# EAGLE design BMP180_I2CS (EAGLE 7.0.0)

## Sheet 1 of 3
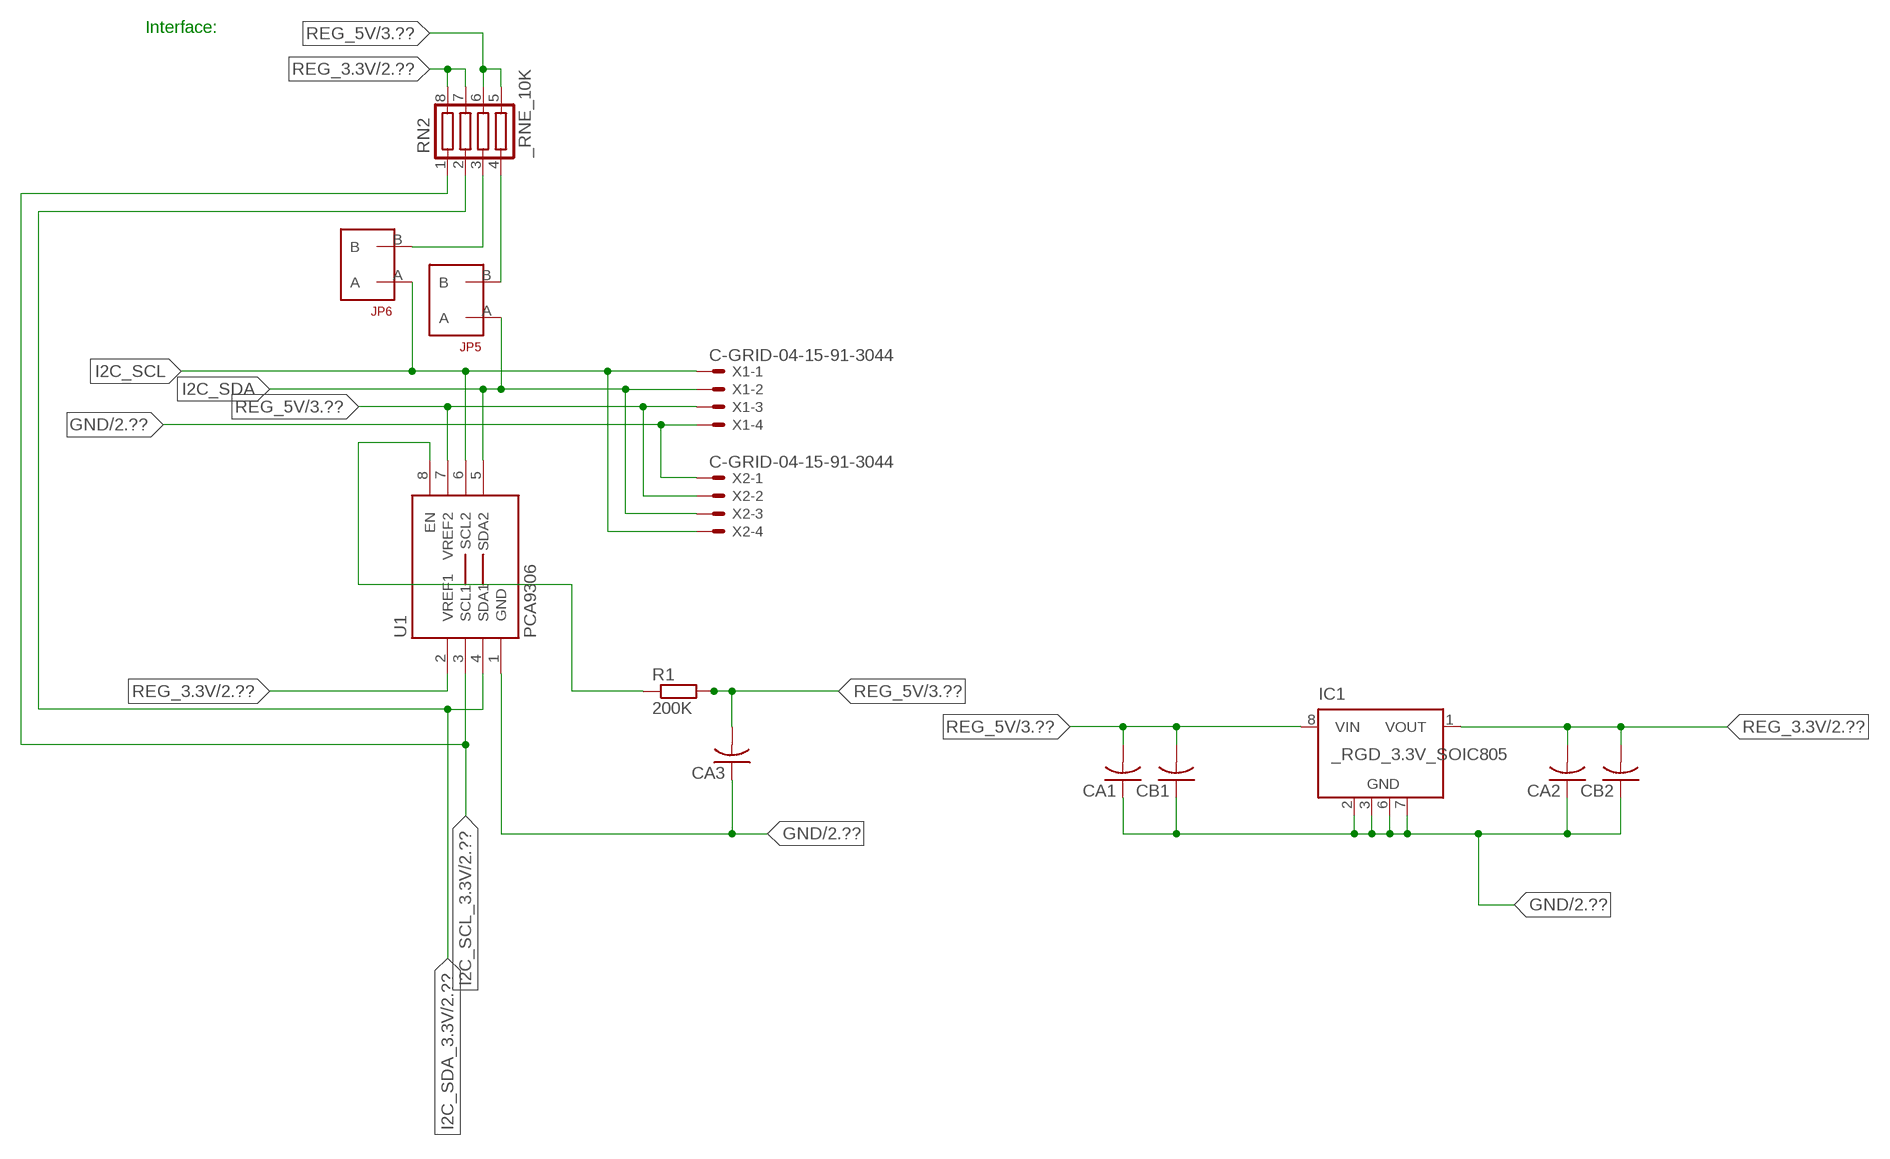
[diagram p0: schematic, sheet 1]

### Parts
CA1  CC1206KRX7R9BB104  [.1UF]
CA2  CC1206KRX7R9BB104  [.1UF]
CA3  CC1206KRX7R9BB104  [.1UF]
CB1  TMK316F106ZL-TC1206K  [TMK316F106ZL-T]
CB2  TMK316F106ZL-TC1206K  [TMK316F106ZL-T]
IC1  _RGD_3.3V_SOIC805  [_RGC_3.3V_SOIC8]
JP5  JUMPER_1X2_2MM  [JUMPER_1X2_2MM]
JP6  JUMPER_1X2_2MM  [JUMPER_1X2_2MM]
R1  200K  RESISTOR_SMT-0603  [R603]
RN2  _RNE_10K  [RNE]
U1  PCA9306  PCA9306_NCD  [PSOP-8]
X1  C-GRID-04-15-91-3044  [15-91-04]
X2  C-GRID-04-15-91-3044  [15-91-04]

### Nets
GND: CA1.1 CA2.1 CA3.1 CB1.1 CB2.1 IC1.2(GND) IC1.3(GND) IC1.6(GND) IC1.7(GND) U1.1(GND) X1.4 X2.1 ; also sheet 2,3
I2C_SCL: JP6.A U1.6(SCL2) X1.1 X2.4
I2C_SCL_3.3V: RN2.1 U1.3(SCL1) ; also sheet 2
I2C_SDA: JP5.A U1.5(SDA2) X1.2 X2.3
I2C_SDA_3.3V: RN2.2 U1.4(SDA1) ; also sheet 2
N$1: JP6.B RN2.3
N$2: JP5.B RN2.4
N$23: R1.1 U1.8(EN)
REG_3.3V: CA2.2 CB2.2 IC1.1(VOUT) RN2.7 RN2.8 U1.2(VREF1) ; also sheet 2
REG_5V: CA1.2 CA3.2 CB1.2 IC1.8(VIN) R1.2 RN2.5 RN2.6 U1.7(VREF2) X1.3 X2.2 ; also sheet 3
Unconnected: IC1.4(NC) IC1.5(NC)

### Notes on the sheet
- Interface:

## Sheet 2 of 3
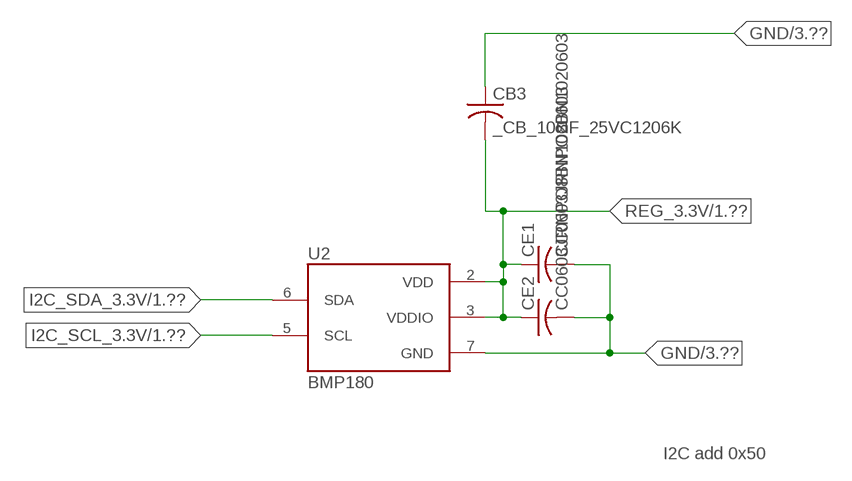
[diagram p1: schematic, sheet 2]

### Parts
CB3  _CB_10UF_25VC1206K  [_CB_10UF_25V]
CE1  CC0603JRNPO8BN1020603  [CC0603JRNPO8BN102]
CE2  CC0603JRNPO8BN1020603  [CC0603JRNPO8BN102]
U2  BMP180  [BMP180]

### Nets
GND: CB3.1 CE1.2 CE2.2 U2.7(GND) ; also sheet 1,3
I2C_SCL_3.3V: U2.5(SCL) ; also sheet 1
I2C_SDA_3.3V: U2.6(SDA) ; also sheet 1
REG_3.3V: CB3.2 CE1.1 CE2.1 U2.2(VDD) U2.3(VDDIO) ; also sheet 1

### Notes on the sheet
- I2C add 0x50

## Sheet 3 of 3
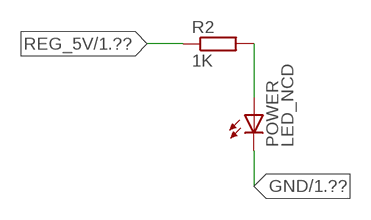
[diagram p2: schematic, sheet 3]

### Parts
POWER  LED_NCD  [CHIPLED_0603]
R2  1K  RESISTOR_SMT-0402  [R402]

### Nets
GND: POWER.C ; also sheet 1,2
N$4: POWER.A R2.2
REG_5V: R2.1 ; also sheet 1

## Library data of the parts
CA1-CA3 = NCD_ULTIMATE_LIBRARY:CC1206KRX7R9BB104: Capacitor CA .1uF 50V SMT C1206K CC1206KRX7R9BB104
CB1 CB2 = NCD_ULTIMATE_LIBRARY:TMK316F106ZL-T: Capacitor CB 10uF SMT 1206 TMK316F106ZL-T
CB3 = NCD_ULTIMATE_LIBRARY:_CB_10UF_25V: Capacitor 10uF SMT
CE1 CE2 = NCD_ULTIMATE_LIBRARY:CC0603JRNPO8BN102: Capacitor CE 1uF SMT CC0603JRNPO8BN102 0603
IC1 = NCD_ULTIMATE_LIBRARY:_RGD_3.3V_SOIC8: Regulator Linear 3.3V Chip Positive VOLTAGE REGULATOR Digikey 497-1199-2-ND/L78L33ACD13TR
JP5 JP6 = NCD_ULTIMATE_CONNECTORS:JUMPER_1X2_2MM
POWER = NCD_ULTIMATE_LIBRARY:LED_NCD: LED Digikey 754-1132-2-ND/APT2012SRCPRV
R1 R2 = NCD_ULTIMATE_LIBRARY:RESISTOR_SMT: NCD Resistor
RN2 = NCD_ULTIMATE_LIBRARY:_RNE_10K: Resistor Array RNE SMT 10K x 4 Single Resistor Source: http://www.ctscorp.com/components/Datasheets/CTSChipArrayDs.pdf Digikey 742C083103JPTR-ND/742C083103JP; OC_FARNELL: unknown; OC_NEWARK: unknown
U1 = NCD_ULTIMATE_LIBRARY:PCA9306_NCD: NCD Bidirectional I2C level shifter. NOT compatible with all available part number pinout schemes- DOUBLE CHECK!!!; PROD_ID: IC-10023
U2 = NCD_ULTIMATE_bhaskar:BMP180: BOSCH BMP180 DIGITAL BAROMETRIC PRESSURE SENSOR Web page: http://www.bosch-sensortec.com/en/homepage/products_3/environmental_sensors_1/bmp180_1/bmp180 Datasheet: http://ae-bst.resource.bosch.com/media/products/dokumente/bmp180/BST-BMP180-DS000-09.pdf The BMP180 is the function compatible successor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
X1 X2 = NCD_ULTIMATE_CONNECTORS:C-GRID-04: CONNECTOR 4-Pos I2C wire to board 2.54 mm (0.100") pitch header Digikey WM1342-ND/0015912045; OC_FARNELL: unknown; OC_NEWARK: unknown

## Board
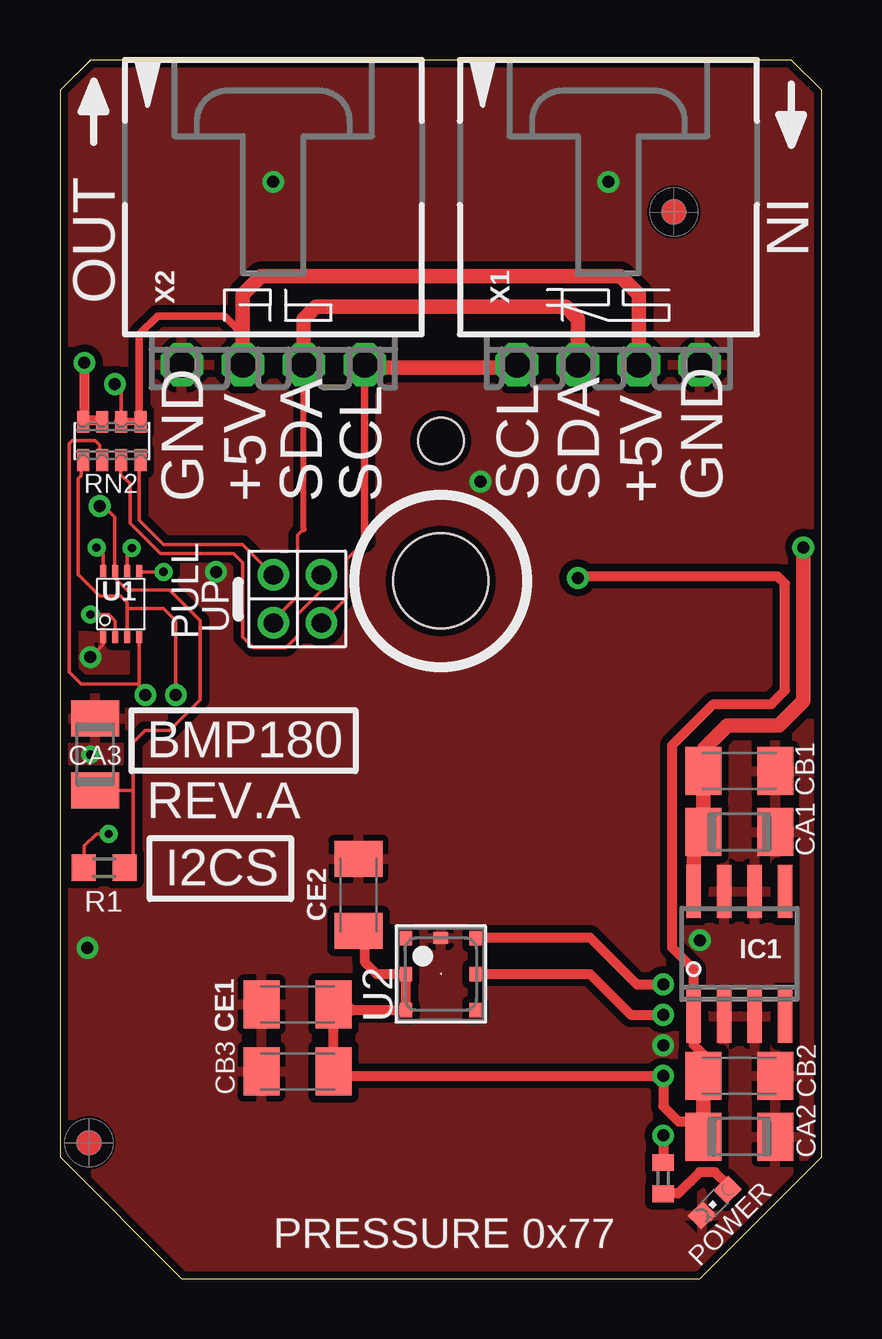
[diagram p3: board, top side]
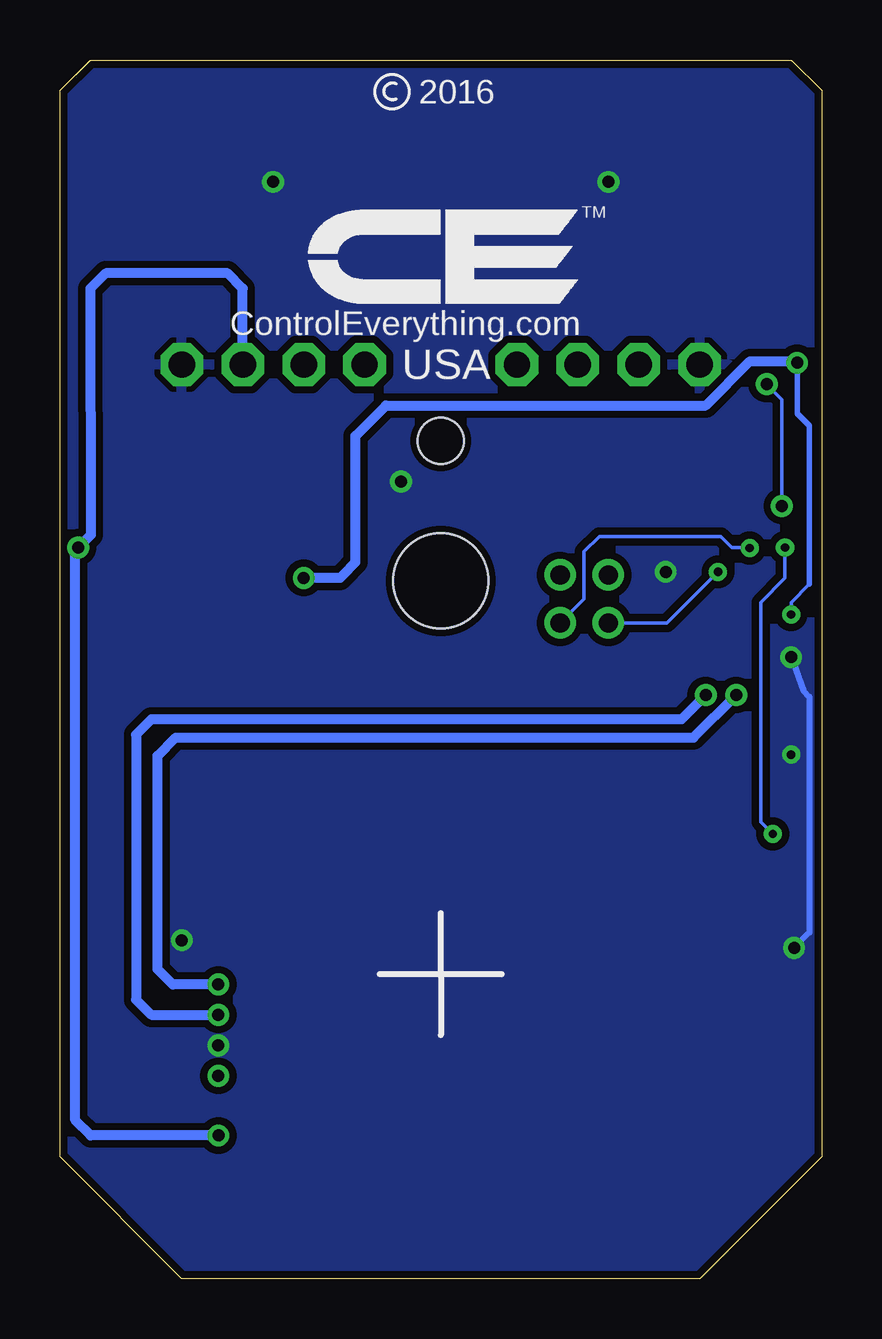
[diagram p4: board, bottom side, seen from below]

Size 31.75 x 50.8 mm. Coordinates in mm from the lower left corner, seen from the top.
Outline: 48 segments
Copper layers (1*16): Top 0.035mm / dielectric 1.5mm / Bottom 0.035mm
Design rules "default": minimum track width 5mil, minimum drill 24mil, track to track 5mil, track to pad 5mil, pad to pad 5mil, via to via 5mil, smd to smd 5mil, copper to edge 10mil, drill to drill 8mil, minimum pad ring 10mil, minimum via ring 8mil, stop-mask expansion 2mil, vias tented up to drill 0mil, thermal gap 10mil
Holes 3.96 mm at 15.88,29.08
Holes 1.91 mm at 15.88,34.93

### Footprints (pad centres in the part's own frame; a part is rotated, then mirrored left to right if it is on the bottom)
.1UF = smd 1.5 x 2: 1 -1.5,0; 2 1.5,0
TMK316F106ZL-T = smd 1.5 x 2: 1 -1.5,0; 2 1.5,0
_CB_10UF_25V = smd 1.5 x 2: 1 -1.5,0; 2 1.5,0
CC0603JRNPO8BN102 = smd 1.5 x 2: 1 -1.5,0; 2 1.5,0
_RGC_3.3V_SOIC8 = smd 0.6 x 2.2: 1 -1.905,-2.6; 2 -0.635,-2.6; 3 0.635,-2.6; 4 1.905,-2.6; 5 1.905,2.6; 6 0.635,2.6; 7 -0.635,2.6; 8 -1.905,2.6
JUMPER_1X2_2MM = drill 0.8: A 0,2; B 0,0
CHIPLED_0603 = smd 0.8 x 0.876: A 0,-0.75; C 0,0.75
R603 = smd 1 x 1.1: 1 -0.85,0; 2 0.85,0
R402 = smd 0.7 x 0.9: 1 -0.65,0; 2 0.65,0
RNE = smd 0.5 x 0.9: 1 -1.2,-0.8; 2 -0.4,-0.8; 3 0.4,-0.8; 4 1.2,-0.8; 5 1.2,0.8; 6 0.4,0.8; 7 -0.4,0.8; 8 -1.2,0.8
PSOP-8 = smd 0.25 x 0.5: 1 -0.73,-1.37; 2 -0.23,-1.37; 3 0.27,-1.37; 4 0.77,-1.37; 5 0.77,1.38; 6 0.27,1.38; 7 -0.23,1.38; 8 -0.73,1.38
BMP180 = smd 0.6 x 0.5: 1 1.5,1.45; 2 0,1.45; 3 -1.5,1.45; 4 -1.5,-1.45; 5 0,-1.45; 6 1.5,-1.45 | smd 0.5 x 0.6: 7 1.5,0
15-91-04 = drill 1.1 pad 1.778 octagon: 1 -3.81,-7.62; 2 -1.27,-7.62; 3 1.27,-7.62; 4 3.81,-7.62

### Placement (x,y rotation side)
CA1  28.32,18.62 180 top
CA2  28.32,5.92 180 top
CA3  1.46,21.86 270 top
CB1  28.32,21.16 180 top
CB2  28.32,8.46 180 top
CB3  9.91,8.64 0 top
CE1  9.91,11.43 180 top
CE2  12.45,16 90 top
IC1  28.32,13.54 0 top
JP5  8.89,29.34 180 top
JP6  10.9,29.34 180 top
POWER  27.3,3.18 135 top
R1  1.84,17.13 0 top
R2  25.15,4.19 270 top
RN2  2.16,34.93 0 top
U1  2.54,28.12 0 top
U2  15.88,12.7 90 top
U$5  [VISION_REF10]  1.21,5.66 90 top
U$28  [VISION_REF10]  25.59,44.46 90 top
X1  22.86,45.72 0 top
X2  8.89,45.72 0 top

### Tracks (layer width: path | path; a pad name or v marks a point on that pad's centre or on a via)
GND  (via drill 0.35, 0.5)
  Top 0.152: CA3.1 1.52,23.42 1.52,23.62 | v1.27,25.91 1.81,26.45 U1.1
  Bottom 0.254: v1.27,25.91 0.76,24.51 0.51,24.26 0.51,14.43 v1.15,13.79
  other vias: 8.89,45.72 22.86,45.72 25.15,9.73 17.53,33.22 26.67,14.11 6.5,29.46 1.27,21.84
  pour Bottom (isolate 0.305): -0.64,5.08 -0.64,49.53 1.27,51.44 30.48,51.44 32.38,49.53 32.38,5.08 26.67,-0.63 5.08,-0.63
  pour Top (isolate 0.305): 4.45,-1.27 -1.27,4.45 -1.27,50.17 0.64,52.07 31.11,52.07 33.02,50.17 33.02,4.45 27.3,-1.27
I2C_SCL  (via drill 0.35)
  Top 0.152: 12.7,30.73 11.94,29.97 11.94,28.38 JP6.A | v3,30.46 2.81,30.24 U1.6
  Top 0.305: 12.7,30.73 X2.4
  Top 0.406: X2.4 12.7,37.97 | 19.05,37.97 X1.1
  Top 0.61: 12.7,37.97 19.05,37.97
  Bottom 0.152: JP6.A 9.91,28.33 9.91,30.3 9.27,30.94 4.19,30.94 3.74,30.48 3.02,30.48 v3,30.46
I2C_SCL_3.3V  (via drill 0.5)
  Top 0.152: RN2.1 0.89,34.07 0.89,33.48 0.77,33.35 0.77,29.35 1.67,28.45 2.54,28.45 2.81,28.18 2.81,27.94 | 2.81,27.94 U1.3 | v4.83,24.33 v4.83,24.34 4.83,27.43 4.32,27.94 2.81,27.94
  Top 0.406: U2.5 22.1,12.7 23.8,11 v25.15,11
  Bottom 0.406: v4.83,24.33 5.84,23.32 27.94,23.32 28.58,22.68 28.58,11.63 27.94,11 v25.15,11
I2C_SDA  (via drill 0.35)
  Top 0.152: JP5.A 8.89,27.44 9.91,28.45 9.91,30.99 10.16,31.24 | U1.5 3.34,29.46 v4.32,29.46
  Top 0.254: 10.16,31.24 10.16,31.25 X2.3
  Top 0.61: X2.3 10.16,40.01 10.67,40.51 21.09,40.51 21.59,40.01 X1.2
  Bottom 0.152: v4.32,29.46 6.45,27.34 JP5.A
I2C_SDA_3.3V  (via drill 0.5)
  Top 0.152: RN2.2 1.65,34.14 1.65,34.75 1.46,34.94 0.51,34.94 0.38,34.81 0.38,26.37 0.38,26.36 0.38,25.3 0.89,24.79 3.31,24.79 | v3.56,24.33 3.31,24.58 3.31,24.79 | 3.31,24.79 U1.4
  Top 0.406: U2.6 17.48,14.22 22.1,14.22 24.05,12.27 v25.15,12.27
  Bottom 0.406: v25.15,12.27 27.05,12.27 27.69,12.9 27.69,21.79 26.93,22.56 5.34,22.56 v3.56,24.33
N$1
  Top 0.152: JP6.B 10.92,29.31 10.92,28.7 9.91,27.69 9.91,26.8 9.42,26.31 8.06,26.31 7.62,26.75 7.62,29.84 7.24,30.23 4.19,30.23 2.92,31.5 2.92,33.15 2.54,33.53 2.54,34.1 RN2.3
  Top 0.305: 2.54,34.02 RN2.3
N$2
  Top 0.152: JP5.B 7.62,30.61 4.32,30.61 3.3,31.62 3.3,34.07 RN2.4
  Top 0.305: 3.37,33.88 RN2.4
N$4
  Top 0.406: POWER.A 27.84,3.92 27.3,4.45 26.67,4.45 25.78,3.56 25.16,3.56 R2.2
N$23  (via drill 0.35)
  Top 0.152: R1.1 1.02,17.16 1.02,18.03 1.52,18.54 v2.03,18.54 | v1.52,30.48 1.81,30.2 U1.8
  Bottom 0.152: v2.03,18.54 2.54,19.05 2.54,28.19 1.52,29.21 v1.52,30.48
REG_3.3V  (via drill 0.35, 0.5)
  Top 0.152: v1.27,27.69 2.03,27.69 2.31,27.41 U1.2
  Top 0.406: CB2.2 26.82,9.35 26.42,9.75 26.42,10.36 | 26.82,6.55 25.78,6.55 25.15,7.19 v25.15,8.46 11.58,8.46 CB3.2 CE1.1 11.94,11.43 12.19,11.18 14.53,11.18 U2.3 U2.2 13.21,12.7 12.7,13.21 12.7,14.25 CE2.1 | IC1.1 26.42,12.9 25.53,13.79 25.53,22.24 27.24,23.95 29.66,23.95 30.23,24.52 30.23,28.97 29.91,29.29 21.67,29.29 v21.59,29.21 | 26.52,5.62 CA2.2 | v1.02,38.18 1.02,35.78 | 1.02,35.78 RN2.8 | 1.02,35.78 1.71,35.78 RN2.7
  Top 0.61: CB2.2 26.82,6.55 CA2.2 | 26.42,10.36 IC1.1
  Bottom 0.152: 0.51,28.96 1.27,28.19 v1.27,27.69
  Bottom 0.229: 0.51,28.96 0.51,35.56 1.02,36.07 v1.02,38.18
  Bottom 0.406: v1.02,38.18 1.08,38.24 2.99,38.24 4.83,36.4 18.16,36.4 19.43,35.13 19.43,29.87 19.94,29.34 20.07,29.21 v21.59,29.21
REG_5V  (via drill 0.5)
  Top 0.152: RN2.6 2.56,37.01 v2.29,37.29 | R1.2 3.05,17.49 3.05,20.36 | 3.05,20.36 3.05,22.35 3.56,22.86 4.57,22.86 5.84,24.13 5.84,27.43 4.57,28.7 2.79,28.7 2.31,29.19 U1.7 2.29,29.52 2.29,31.75 1.83,32.21 v1.65,32.21 | CA3.2 3.05,20.36
  Top 0.305: 7.62,39.37 7.5,39.37 | 2.42,35.74 RN2.6 RN2.5 3.31,35.8 3.31,39.37 4.07,40.13 6.86,40.13 7.62,39.37 | X2.2 7.62,39.37
  Top 0.406: v25.15,5.97 R2.1
  Top 0.61: X2.2 7.62,41.02 8.38,41.78 23.37,41.78 24.13,41.02 X1.3 | IC1.8 26.42,18.21 CA1.2 CB1.2 26.86,21.2 26.86,22.11 27.82,23.06 29.98,23.06 30.99,24.08 v30.99,30.48
  Bottom 0.152: v1.65,32.21 1.65,36.65 v2.29,37.29
  Bottom 0.406: X1.3 24.13,41.28 24.77,41.91 29.84,41.91 30.48,41.27 30.47,31 v30.99,30.48 31.11,30.36 31.11,6.6 30.48,5.97 v25.15,5.97

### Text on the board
tNames: IN | OUT | GND | +5V | SDA | SCL | SCL | SDA | +5V | GND | PULL | UP | BMP180 | REV.A | I2CS | PRESSURE 0x77
bNames: 2016 | TM | ControlEverything.com | USA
